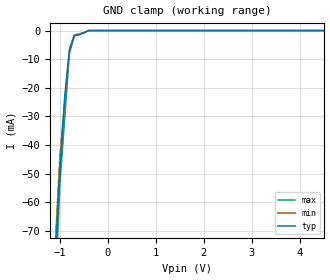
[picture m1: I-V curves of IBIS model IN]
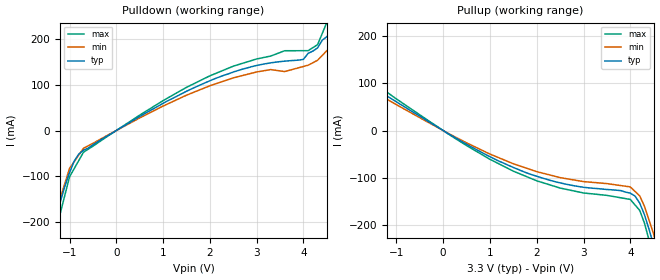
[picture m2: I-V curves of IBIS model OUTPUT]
|   PERICOM SEMICONDUCTOR CORP
|   IBIS Model of PI6CV304
|   Product Family: 6CV
|   TSSOP (L) Package
[IBIS Ver] 3.2
[Comment char] |_char
[File Name] pi6cv304_l_reva.ibs
[File Rev] 2.0
[Source] File originated at Pericom Semiconductor Corp.
[Date] 10/08/12
[Disclaimer] (C) Copyright PERICOM Semiconductor Corporation
   All rights reserved
  Pericom Semiconductor Corporation hereby grants the user of
  this IBIS model a non-exclusive, nontransferable license to
  use this IBIS model under the following terms.
  This IBIS model is provided on an "AS IS" basis and Pericom
  makes absolutely no warranty with respect to the information
  contained herein. PERICOM DISCLAIMS AND CUSTOMER WAIVES ALL
  WARRANTIES, EXPRESSED OR IMPLIED, INCLUDING WARRANTIES OF
  MERCHANTABILITY OR FITNESS FOR A PARTICULAR PURPOSE. The
  entire risk as to quality and performance is with the customer.
  Accordingly, in no event shall the company be liable for any
  damages, whether in contract or tort, including any lost
  profits or other incidental, consequential, exemplary, or
  punitive damages arising out of the use or application of the
  IBIS model provided in this package. Further, Pericom reserves
  the right to make changes without notice to any product herein
  to improve reliability, function, or design. Pericom does not
  convey any license under patent rights or any other intellectual
  property rights, including those of third parties.
  The user is granted this license only to use the IBIS model
  and is not granted rights to sell, load, rent, lease or license
  the IBIS model in whole or in part, or in modified form to anyone
  other than user. User may modify the IBIS model to suit its specific
  application but rights to derivative works and such modifications
  shall belong to Pericom.
  Pericom is not obligated to provide maintenance or support
  for the licensed IBIS model.
  Contact Pericom at ATTN: APPLICATION ENGINEERING / IBIS MODELS
  1545 Barber Lane Milpitas, CA 95035 USA.
[Component] PI6CV304
[Manufacturer] Pericom Semiconductor Corp.
[Package]
| variable   typ   min   max
R_pkg   0.05434ohm   0.05089ohm   0.05779ohm
L_pkg   2.52412nH   2.40183nH   2.64640nH
C_pkg   0.18313pF   0.16762pF   0.19864pF
[Pin] signal_name   model_name   R_pin   L_pin   C_pin
1   CLK_IN   IN   0.05089   2.64640nH   0.19864pF
2   OE   IN   0.05779   2.40183nH   0.16762pF
3   Y0   OUTPUT   0.05779   2.40183nH   0.16762pF
4   GND   GND   0.05089   2.64640nH   0.19864pF
5   Y1   OUTPUT   0.05089   2.64640nH   0.19864pF
6   VDD   POWER   0.05779   2.40183nH   0.16762pF
7   Y2   OUTPUT   0.05779   2.40183nH   0.16762pF
8   Y3   OUTPUT   0.05089   2.64640nH   0.19864pF
| Models and submodels in the file (2): IN (Input), OUTPUT (Output)
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|   Model CLK_IN
[Model] IN
Model_type Input
Vinl = 800mV
Vinh = 2.00V
| variable   typ   min   max
C_comp   5.000pF   4.75pF   5.25pF
[Voltage Range]   3.300V   3.15   3.45
[GND Clamp Reference]   0.000V   0   0
[POWER Clamp Reference]   3.300V   3.15   3.45
[Temperature Range]   25.00   85.00   -45.000
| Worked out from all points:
|   GND clamp passes 1 mA (typ) near -0.53 V on its own axis
[GND Clamp]
| Voltage   I(typ)   I(min)   I(max)
| Voltage   I(typ)   I(min)   I(max)
-3.3V     -971.4mA   -874.3mA   -1.069A
-1.101V   -80.64mA   NA         NA
-999.6mV  -48.85mA   -43.96mA   -53.73mA
-898.5mV  -23.02mA   NA         NA
-802.5mV  -7.31mA    -6.579mA   -8.041mA
-701.1mV  -1.74mA    -1.566mA   -1.914mA
-599.9mV  -1.43mA    NA         NA
-402.9mV  0A         0A         0A
6.602V    0A         0A         0A
[POWER Clamp]   |Note: Vtable = Vcc - Voutput
| Voltage   I(typ)   I(min) I(max)
-3.3V     0A         NA         NA
0V        0A         NA         NA
|   Model OUTPUT
[Model] OUTPUT
Model_type Output
Polarity   Non-Inverting
Vref = 0.00V
Rref = 500ohms
Vmeas = 1.65V
| variable   typ   min   max
C_comp   6.000pF  5.5pF   6.3pF
[Voltage Range]   3.300V   3.15   3.45
[POWER Clamp Reference]   3.300V   NA   NA
[GND Clamp Reference]   0.000V   NA   NA
[Pullup Reference]   3.300V   NA   NA
[Pulldown Reference]   0.000V   NA   NA
[Temperature Range]   25.00   85.00  -45.000
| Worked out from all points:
|   slope of the pulldown table from 0 to 0.495 V, typ, clamps not added: 16.3 ohm
|   slope of the pullup table from 0 to 0.495 V, typ, clamps not added: 17.3 ohm
[Pulldown]
| Voltage   I(typ)   I(min)  I(max)
-3.3V     -970.1mA   -873.1mA   -1.067A
-1.5V     -275.4mA   -247.9mA   -302.9mA
-1.399V   -233.1mA   NA         NA
-1.303V   -195.7mA   NA         NA
-999.7mV  -92.08mA   -82.87mA   -101.3mA
-701.1mV  -43.09mA   -38.78mA   -47.4mA
2.001V    108.7mA    97.87mA    119.6mA
4.099V    168.7mA    142.8mA    174.5mA
4.301V    180.6mA    153.5mA    187.7mA
4.499V    205.3mA    174.5mA    236.1mA
5.101V    265.9mA    NA         NA
6.602V    864.3mA    734.7mA    994mA
[Pullup]   |Note: Vtable = Vcc - Voutput
| Voltage   I(typ)   I(min)   I(max)
-3.3V     222.2mA    200mA      244.4mA
-2.901V   201.6mA    NA         NA
-2.8V     194.9mA    NA         NA
-1.5V     92.51mA    83.26mA    101.8mA
99.58mV   -6.14mA    -5.526mA   -6.754mA
1.202V    -65.12mA   NA         NA
2.501V    -110.4mA   -99.4mA    -121.5mA
3.998V    -132.2mA   -119mA     -145.4mA
4.2V      -153.2mA   -137.9mA   -168.5mA
4.402V    -209.4mA   NA         NA
4.499V    -243mA     -218.7mA   -267.3mA
6.603V    -1.056A    -950.8mA   -1.162A
[Ramp]
| variable   typ   min   max
dV/dt_r   1.98/527.00p   1.98/560.00p   1.98/490p
dV/dt_f   1.98/457.00p   1.98/480.00p   1.98/500.00p
R_load = 500ohms
